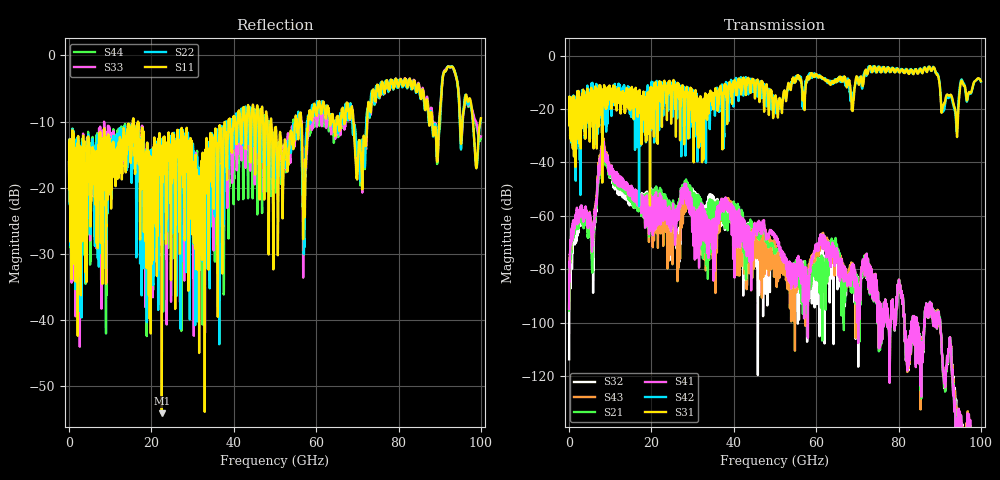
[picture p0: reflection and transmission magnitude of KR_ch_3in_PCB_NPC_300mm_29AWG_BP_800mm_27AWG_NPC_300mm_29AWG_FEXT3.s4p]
# GHz S RI R 45
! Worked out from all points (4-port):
!   4000 points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, 25 MHz to 100 GHz, reference 45 ohm
!   strongest paths, dB at 25 MHz, 25.02 GHz, 50.02 GHz, 75.03 GHz, 100 GHz:
!     S31: -20.7, -14.9, -15.6, -5.1, -9.6
!     S42: -20.6, -18.0, -18.0, -4.3, -9.8
!     S41: -94.8, -60.5, -67.0, -90.5, -147.7
!     S21: -95.5, -56.8, -74.0, -90.6, -153.0
!     S43: -94.9, -71.8, -71.3, -90.4, -153.9
!     S32: -113.8, -64.5, -77.5, -90.5, -154.8
!   lowest |S11| = -54.1 dB at 22.52 GHz (marker M1), VSWR 1.00, Z = 44.9 + j0.162 ohm
!   |S11| at or under -10 dB: start of sweep to 15.52 GHz; 16.75 GHz to 38.73 GHz (21.98 GHz wide, 79.2 % of centre); 49.11 GHz to 54.97 GHz (5.854 GHz wide, 11.2 % of centre)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
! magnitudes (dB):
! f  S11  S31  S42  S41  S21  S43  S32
! 25 MHz  -16.1  -20.7  -20.6  -94.8  -95.5  -94.9  -113.8
! 5.775 GHz  -14.8  -26.9  -20.4  -68.9  -73.2  -68.0  -75.1
! 8.225 GHz  -14.4  -13.5  -21.1  -32.9  -34.8  -31.6  -33.2
! 22.52 GHz  -54.1  -23.3  -11.1  -60.9  -55.9  -66.5  -60.2
! 38.65 GHz  -11.9  -14.9  -14.6  -55.2  -59.9  -53.7  -57.2
! 54.15 GHz  -12.4  -9.5  -9.8  -79.0  -79.8  -83.5  -84.9
! 100 GHz  -9.5  -9.6  -9.8  -147.7  -153.0  -153.9  -154.8
